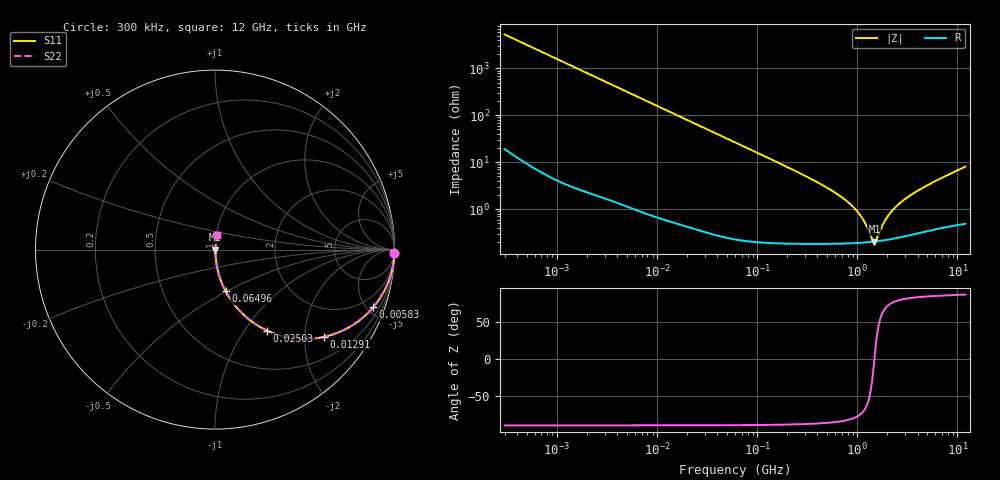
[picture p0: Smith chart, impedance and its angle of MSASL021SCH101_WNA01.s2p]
! MSASL021SCH101_WNA01  S-PARAMETER MODEL  ( Standard Model )
! Model Generated by TAIYO YUDEN Corporation (http://www.ty-top.com)
! Version 4.0
! TAIYO YUDEN Control No. 240513
! Copyright(c) 2017 TAIYO YUDEN CO.,LTD. All Rights Reserved.
! Product Description (link to TY-COMPAS)
! https://ds.yuden.co.jp/TYCOMPAS/or/detail?pn=MSASL021SCH101JWNA01&u=M
! Products Name : Multilayer Ceramic Capacitors
! Characteristics :
!  Capacitance : 100 [pF] , Rated Voltage : 10 [V] , TCC : CH / C0H
!  Case Size : 0.25 x 0.125 / 0.0098 x 0.0049 [mm/inch] , Thickness : 0.125 / 0.0049 [mm/inch]
!  (Conditions: Temperature = 25 [degC] , DC Bias Voltage = 0 [V])
! External Node Assignments :
!  1  o---| |---o  2
! GND o---------o GND
! Frequency Range : 0.3MHz  -  12000MHz  [ 401 STEP ]
# MHZ S RI R 50
! Freq[MHz].  S11 Real  S11 Imag  S21 Real  S21 Imag  S12 Real  S12 Imag  S22 Real  S22 Imag
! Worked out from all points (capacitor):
!   401 points, 300 kHz to 12 GHz, reference 50 ohm
!   read as one part in series: C = 100 pF near 316.3 kHz
!   lowest |Z| = 203 mohm at 1.48 GHz (marker M1)
!   series resonance near 1.482 GHz, so ESL is about 120 pH
!   S11 on the Smith chart (normalised r, x): 300 kHz: open; 5.83 MHz: 1.02, -5.48; 12.91 MHz: 1.01, -2.48; 25.03 MHz: 1.01, -1.28; 64.96 MHz: 1.00, -0.49; 12 GHz: 1.01, +0.16
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0.3  0.9996 -0.0189  0.000424 0.0189  0.000424 0.0189  0.9996 -0.0189
1.769972  0.9875 -0.1097  0.0125 0.1097  0.0125 0.1097  0.9875 -0.1097
5.830396  0.8814 -0.3215  0.1186 0.3215  0.1186 0.3215  0.8814 -0.3215
10.44266  0.7001 -0.4561  0.2999 0.4561  0.2999 0.4561  0.7001 -0.4561
12.90781  0.605 -0.4866  0.395 0.4866  0.395 0.4866  0.605 -0.4866
25.03118  0.2915 -0.4516  0.7085 0.4516  0.7085 0.4516  0.2915 -0.4516
38.24403  0.151 -0.3547  0.849 0.3547  0.849 0.3547  0.151 -0.3547
60  0.0683 -0.2481  0.9317 0.2481  0.9317 0.2481  0.0683 -0.2481
64.96309  0.0591 -0.2314  0.9409 0.2314  0.9409 0.2314  0.0591 -0.2314
140.0606  0.0145 -0.1117  0.9855 0.1117  0.9855 0.1117  0.0145 -0.1117
353.9943  0.00362 -0.0425  0.9964 0.0425  0.9964 0.0425  0.00362 -0.0425
617.4538  0.00228 -0.0214  0.9977 0.0214  0.9977 0.0214  0.00228 -0.0214
894.6982  0.002 -0.0113  0.998 0.0113  0.998 0.0113  0.002 -0.0113
1105.905  0.00196 -0.00638  0.998 0.00638  0.998 0.00638  0.00196 -0.00638
1403.667  0.00201 -0.00116  0.998 0.00116  0.998 0.00116  0.00201 -0.00116
1480.043  0.00203 -2.33e-05  0.998 2.33e-05  0.998 2.33e-05  0.00203 -2.33e-05
1560.575  0.00206 0.00111  0.9979 -0.00111  0.9979 -0.00111  0.00206 0.00111
1829.429  0.00217 0.00454  0.9978 -0.00454  0.9978 -0.00454  0.00217 0.00454
2088.533  0.00231 0.00746  0.9977 -0.00746  0.9977 -0.00746  0.00231 0.00746
2650.866  0.00265 0.013  0.9973 -0.013  0.9973 -0.013  0.00265 0.013
3740.715  0.00343 0.0222  0.9966 -0.0222  0.9966 -0.0222  0.00343 0.0222
12000  0.0112 0.0792  0.9888 -0.0792  0.9888 -0.0792  0.0112 0.0792
